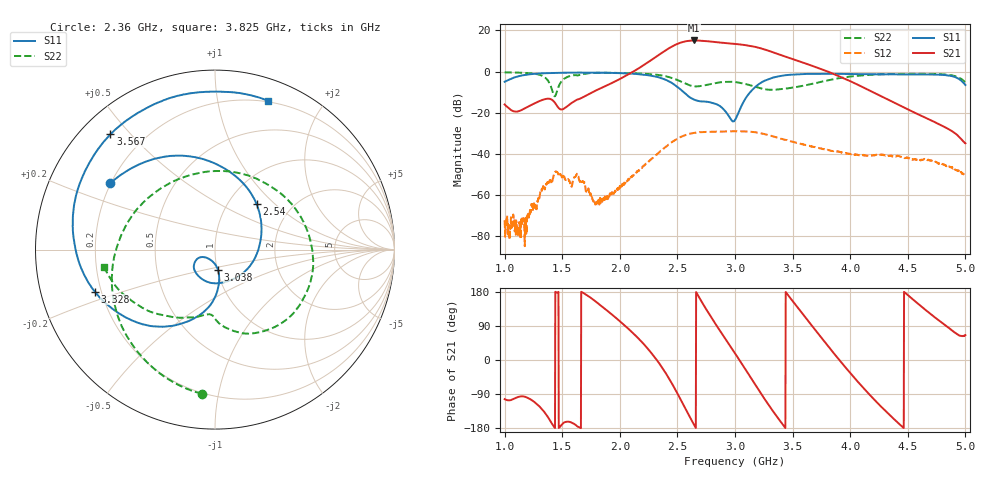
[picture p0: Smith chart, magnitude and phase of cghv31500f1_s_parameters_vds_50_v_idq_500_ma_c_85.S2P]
!Keysight Technologies,E5071C,MY46632031,B.14.03
!Date: Fri Jul 09 16:45:14 2021
!Data & Calibration Information:
!Freq	S11:SOLT2(ON)	S21:SOLT2(ON)	S12:SOLT2(ON)	S22:SOLT2(ON)
!PortZ  Port1:50+j0  Port2:50+j0
!Above PortZ is port z conversion or system Z0 setting when saving the data.
!When reading, reference impedance value at option line is always used.
# Hz S dB R 50
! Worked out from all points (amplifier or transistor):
!   1601 points, 1 GHz to 5 GHz, reference 50 ohm
!   highest |S21| = 15.1 dB at 2.645 GHz (marker M1)
!   |S21| within 3 dB of that: 2.451 GHz to 3.167 GHz (715.8 MHz wide, 25.5 % of centre)
!   unconditionally stable (mu >= 1): start of sweep to end of sweep
!   at 1.665 GHz: K = 34.10, MAG = 2.2 dB, |S12| = -53.9 dB
!   at 3 GHz: K = 2.16, MAG = 15.1 dB, |S12| = -29.0 dB
!   at 5 GHz: K = 5043.35, MAG = -32.2 dB, |S12| = -50.5 dB
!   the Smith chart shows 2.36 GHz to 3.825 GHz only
!   S11 on the Smith chart (normalised r, x): 2.36 GHz: 0.20, +0.28; 2.54 GHz: 1.35, +0.78; 3.038 GHz: 1.01, -0.23; 3.328 GHz: 0.17, -0.16; 3.567 GHz: 0.08, +0.44; 3.825 GHz: 0.19, +1.40
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1e9  -4.98 153.6  -15.97 -103.3  -72.20 130.5  -0.39 122.0
1.3125e9  -0.91 75.5  -14.10 -125.7  -57.88 -120.6  -1.75 62.2
1.6675e9  -0.50 -14.7  -12.82 179.6  -53.62 -165.0  -1.43 54.6
2.06e9  -0.90 -112.8  -1.83 86.4  -52.72 2.3  -0.72 -19.8
2.335e9  -2.78 158.3  7.94 -5.8  -39.47 -88.0  -1.66 -86.9
2.36e9  -3.21 147.7  8.88 -16.7  -38.33 -99.4  -1.87 -95.3
2.45e9  -5.47 103.7  12.06 -60.7  -34.39 -143.1  -3.08 -131.1
2.54e9  -9.28 47.7  14.23 -111.2  -31.49 166.2  -5.12 -178.6
2.645e9  -13.61 -32.8  15.09 -171.1  -29.76 106.3  -7.16 111.6
2.715e9  -14.52 -80.6  14.94 151.5  -29.37 69.1  -6.91 66.9
2.8125e9  -15.35 -125.9  14.41 103.6  -29.23 21.3  -5.76 18.4
2.8975e9  -18.11 -150.1  13.92 64.3  -29.12 -17.7  -5.06 -13.9
3e9  -23.53 -103.3  13.39 17.6  -28.98 -64.5  -5.11 -46.1
3.0375e9  -18.99 -81.6  13.19 0.2  -28.95 -81.6  -5.42 -56.3
3.18e9  -7.30 -111.3  11.92 -67.1  -29.46 -148.5  -7.49 -85.1
3.3275e9  -2.98 -160.8  9.39 -134.1  -31.40 144.6  -8.83 -95.4
3.5675e9  -1.24 132.2  4.76 129.2  -35.03 49.4  -7.15 -120.6
3.6675e9  -1.10 107.8  2.84 90.5  -36.26 12.2  -5.97 -137.1
3.825e9  -1.11 70.6  -0.44 30.2  -38.25 -43.7  -4.07 -171.0
4.335e9  -1.39 -61.2  -13.83 -143.0  -40.90 175.9  -1.23 65.2
4.705e9  -1.43 -162.9  -23.77 119.8  -43.06 89.5  -1.12 -0.1
5e9  -6.54 124.8  -34.81 65.7  -50.49 33.7  -5.29 -43.6
